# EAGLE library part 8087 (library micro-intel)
MICROCOMPUTER/PERIPHERAL DEVICE
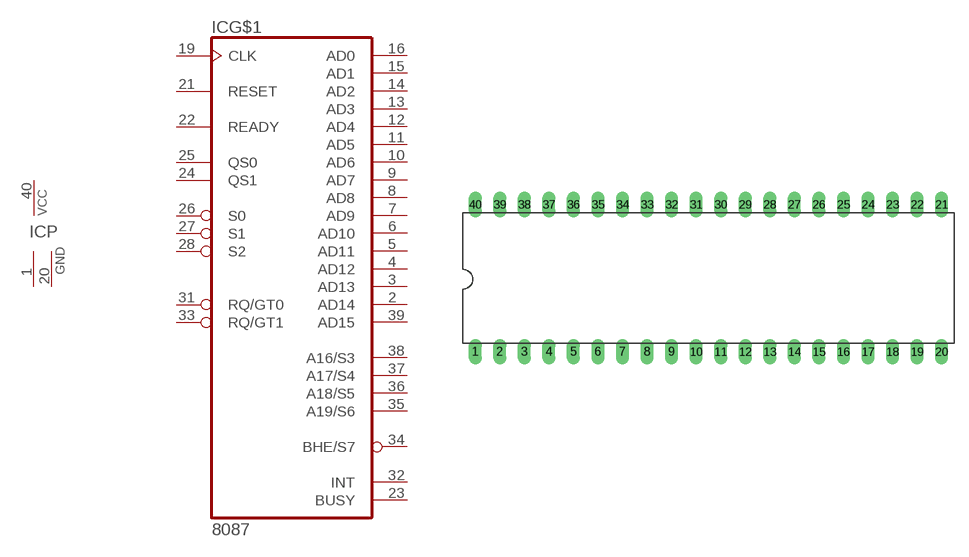
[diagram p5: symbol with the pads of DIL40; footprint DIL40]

Designator prefix IC; gates G$1=8087 P=PWR2GND

## 8087 (OC_FARNELL: unknown; OC_NEWARK: unknown)  [DIL40]
1  P:GND  pwr
2  G$1:AD14
3  G$1:AD13
4  G$1:AD12
5  G$1:AD11
6  G$1:AD10
7  G$1:AD9
8  G$1:AD8
9  G$1:AD7
10  G$1:AD6
11  G$1:AD5
12  G$1:AD4
13  G$1:AD3
14  G$1:AD2
15  G$1:AD1
16  G$1:AD0
19  G$1:CLK  in
20  P:GND  pwr
21  G$1:RESET  in
22  G$1:READY  in
23  G$1:BUSY  out
24  G$1:QS1  in
25  G$1:QS0  in
26  G$1:S0
27  G$1:S1
28  G$1:S2
31  G$1:RQ/GT0
32  G$1:INT  out
33  G$1:RQ/GT1
34  G$1:BHE/S7
35  G$1:A19/S6
36  G$1:A18/S5
37  G$1:A17/S4
38  G$1:A16/S3
39  G$1:AD15
40  P:VCC  pwr

## Footprint DIL40 (pad centres in mm)
Dual In Line Package
drill 0.813 long: 1 -24.13,-7.62; 2 -21.59,-7.62; 3 -19.05,-7.62; 4 -16.51,-7.62; 5 -13.97,-7.62; 6 -11.43,-7.62; 7 -8.89,-7.62; 8 -6.35,-7.62; 9 -3.81,-7.62; 10 -1.27,-7.62; 11 1.27,-7.62; 12 3.81,-7.62; 13 6.35,-7.62; 14 8.89,-7.62; 15 11.43,-7.62; 16 13.97,-7.62; 17 16.51,-7.62; 18 19.05,-7.62; 19 21.59,-7.62; 20 24.13,-7.62; 21 24.13,7.62; 22 21.59,7.62; 23 19.05,7.62; 24 16.51,7.62; 25 13.97,7.62; 26 11.43,7.62; 27 8.89,7.62; 28 6.35,7.62; 29 3.81,7.62; 30 1.27,7.62; 31 -1.27,7.62; 32 -3.81,7.62; 33 -6.35,7.62; 34 -8.89,7.62; 35 -11.43,7.62; 36 -13.97,7.62; 37 -16.51,7.62; 38 -19.05,7.62; 39 -21.59,7.62; 40 -24.13,7.62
